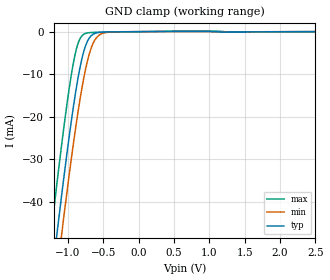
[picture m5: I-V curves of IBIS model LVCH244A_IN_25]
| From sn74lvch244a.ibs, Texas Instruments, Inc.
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[Model]   LVCH244A_IN_25
Model_type  Input
Vinl=0.7
Vinh=1.7
| variable   typ   min   max
C_comp   3.45pF   3.08pF   4.07pF
[Temperature Range]   40   100   -40
| Ambient temperature   25   85   -40
[Voltage range]   2.5   2.3   2.7
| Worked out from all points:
|   GND clamp passes 1 mA (typ) near -0.67 V on its own axis
[GND Clamp]
| LVCH244A_IN_25
|   Voltage   I(typ)   I(min)   I(max)
-5.5V     -732.9mA   -739.4mA   -725.3mA
-1.245V   -60.26mA   -69.5mA    -48.42mA
-1.165V   -48.91mA   -58.17mA   -37mA
-1.14V    -45.44mA   -54.7mA    -33.52mA
-1.095V   -39.28mA   -48.52mA   -27.4mA
-1.075V   -36.59mA   -45.81mA   -24.75mA
-955mV    -21.38mA   -30.25mA   -10.43mA
-865mV    -11.63mA   -19.7mA    -3.173mA
-740mV    -2.841mA   -8.001mA   -359.1uA
-650mV    -685.4uA   -2.964mA   -189.7uA
-565mV    -206.6uA   -904.5uA   -150.9uA
2.5V      1.117nA    83.8nA     -473.3pA
